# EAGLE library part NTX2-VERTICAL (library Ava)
Radiometrix NTX2 Transmitter Module Author Anthony Stirk / http://ava.upuaut.net
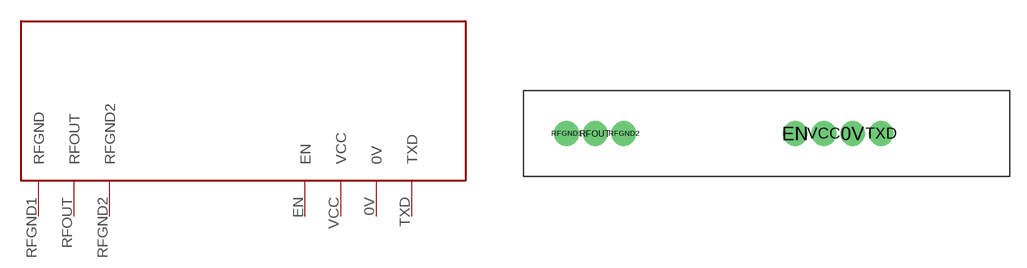
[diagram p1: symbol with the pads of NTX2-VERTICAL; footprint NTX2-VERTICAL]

Designator prefix -

## NTX2-VERTICAL  [NTX2-VERTICAL]
0V  0V
EN  EN
RFGND1  RFGND
RFGND2  RFGND2
RFOUT  RFOUT
TXD  TXD
VCC  VCC

## Footprint NTX2-VERTICAL (pad centres in mm)
Radiometrix NTX2 http://www.radiometrix.com/files/additional/ntx2nrx2.pdf Vertical mounted orientation
drill 0.7 pad 2.184: 0V 17.78,0; EN 12.7,0; RFGND1 -7.62,0; RFGND2 -2.54,0; RFOUT -5.08,0; TXD 20.32,0; VCC 15.24,0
